FUNCTION_BLOCK FB_DO_IED_LD1_MMXU1_PhV EXTENDS FB_AcsiCommonDataClass
VAR_INPUT
	phsA: FB_DO_IED_LD1_MMXU1_PhV_phsA := (sClass:='CMV', bLinkResult:=THIS^.AddDataToContainer(ipData:=phsA));
END_VAR
VAR
END_VAR

END_FUNCTION_BLOCK
